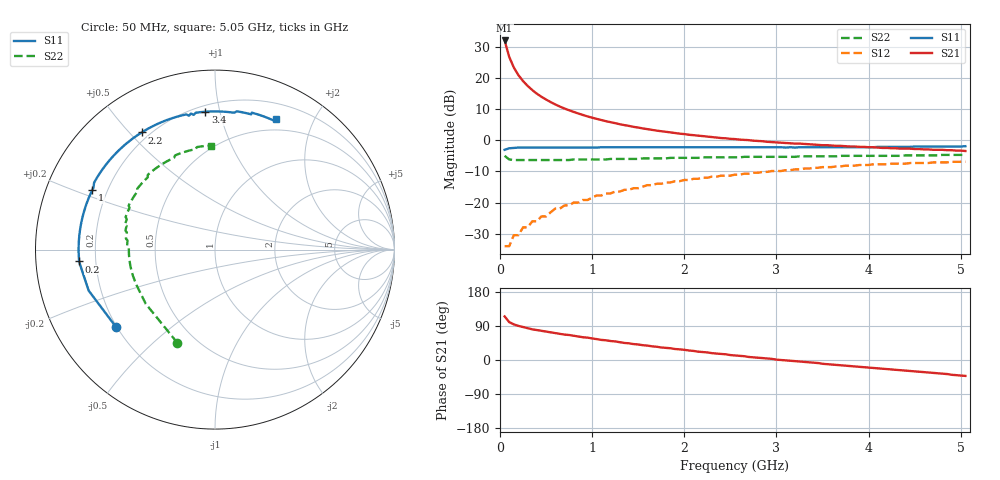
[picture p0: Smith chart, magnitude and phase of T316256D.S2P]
!AT-31625
!S-PARAMETERS at Vce=6.0 V  Ic=200 mA.  LAST UPDATED 08-05-96
# ghz s ma r 50
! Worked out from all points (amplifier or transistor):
!   101 points, 50 MHz to 5.05 GHz, reference 50 ohm
!   highest |S21| = 31.9 dB at 50 MHz (marker M1)
!   |S21| within 3 dB of that: start of sweep to 78.42 MHz
!   unconditionally stable (mu >= 1): 397.2 MHz to 410.7 MHz; 464 MHz to 599.5 MHz; 600.2 MHz to 1.562 GHz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
!   at 850 MHz: K = 1.05, MAG = 12.8 dB, |S12| = -20.0 dB
!   at 2.55 GHz: K = 0.96, MSG = 5.7 dB, |S12| = -11.1 dB
!   at 5.05 GHz: K = 0.94, MSG = 1.7 dB, |S12| = -6.9 dB
!   S11 on the Smith chart (normalised r, x): 50 MHz: 0.20, -0.33; 200 MHz: 0.14, -0.04; 1 GHz: 0.14, +0.23; 2.2 GHz: 0.17, +0.54; 3.4 GHz: 0.24, +0.90; 5.05 GHz: 0.37, +1.50
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0.05  0.7 -142.0  39.55 115.0  0.02 41.0  0.56 -112.0
0.1  0.74 -162.0  21.54 100.0  0.02 43.0  0.49 -142.0
0.15  0.75 -171.0  14.58 94.0  0.03 48.0  0.48 -156.0
0.2  0.76 -175.0  11 90.0  0.03 53.0  0.48 -162.0
0.25  0.76 -179.0  8.84 87.0  0.04 56.0  0.48 -166.0
0.3  0.76 178.0  7.39 84.0  0.04 59.0  0.48 -169.0
0.35  0.76 176.0  6.35 81.0  0.05 61.0  0.48 -171.0
0.4  0.76 174.0  5.55 79.0  0.05 62.0  0.48 -173.0
0.45  0.76 172.0  4.95 77.0  0.06 63.0  0.48 -175.0
0.5  0.76 170.0  4.47 75.0  0.06 63.0  0.48 -176.0
0.6  0.76 166.0  3.73 71.0  0.08 64.0  0.48 -178.0
0.7  0.76 163.0  3.21 67.0  0.09 64.0  0.48 -180.0
0.9  0.76 157.0  2.53 60.0  0.11 62.0  0.49 177.0
1  0.76 154.0  2.29 57.0  0.12 61.0  0.49 176.0
1.1  0.77 151.0  2.1 53.0  0.13 60.0  0.49 174.0
1.35  0.77 144.0  1.74 45.0  0.16 56.0  0.5 171.0
1.75  0.77 134.0  1.39 33.0  0.2 50.0  0.51 166.0
2.2  0.77 122.0  1.16 21.0  0.25 42.0  0.53 160.0
2.55  0.77 114.0  1.04 12.0  0.28 36.0  0.53 155.0
3.4  0.77 94.0  0.85 -7.0  0.36 21.0  0.55 139.0
4.25  0.78 79.0  0.74 -25.0  0.42 3.0  0.56 117.0
5.05  0.8 65.0  0.67 -42.0  0.45 -14.0  0.58 92.0
